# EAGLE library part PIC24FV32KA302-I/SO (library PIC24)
16-bit Microcontrollers a,SOIC-28
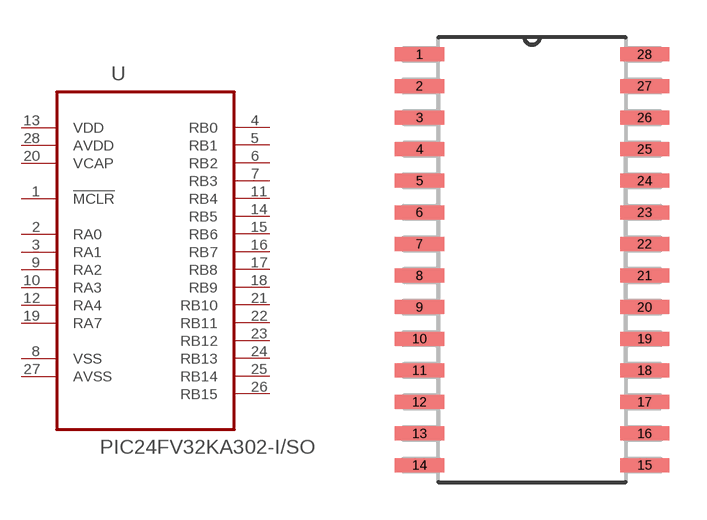
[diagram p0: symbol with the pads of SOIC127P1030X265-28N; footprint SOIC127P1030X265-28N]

Designator prefix U

## PIC24FV32KA302-I/SO (MPN: PIC24FV32KA302-I/SO; OC_FARNELL: 1898815; OC_NEWARK: 13T4818; PACKAGE: SOIC-28; SUPPLIER: MICROCHIP)  [SOIC127P1030X265-28N]
1  !MCLR  in
2  RA0
3  RA1
4  RB0
5  RB1
6  RB2
7  RB3
8  VSS  pas
9  RA2
10  RA3
11  RB4
12  RA4
13  VDD  pwr
14  RB5
15  RB6
16  RB7
17  RB8
18  RB9
19  RA7
20  VCAP  pwr
21  RB10
22  RB11
23  RB12
24  RB13
25  RB14
26  RB15
27  AVSS  pas
28  AVDD  pwr

## Footprint SOIC127P1030X265-28N (pad centres in mm)
smd 1.981 x 0.559: 1 -4.521,8.255; 2 -4.521,6.985; 3 -4.521,5.715; 4 -4.521,4.445; 5 -4.521,3.175; 6 -4.521,1.905; 7 -4.521,0.635; 8 -4.521,-0.635; 9 -4.521,-1.905; 10 -4.521,-3.175; 11 -4.521,-4.445; 12 -4.521,-5.715; 13 -4.521,-6.985; 14 -4.521,-8.255; 15 4.521,-8.255; 16 4.521,-6.985; 17 4.521,-5.715; 18 4.521,-4.445; 19 4.521,-3.175; 20 4.521,-1.905; 21 4.521,-0.635; 22 4.521,0.635; 23 4.521,1.905; 24 4.521,3.175; 25 4.521,4.445; 26 4.521,5.715; 27 4.521,6.985; 28 4.521,8.255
